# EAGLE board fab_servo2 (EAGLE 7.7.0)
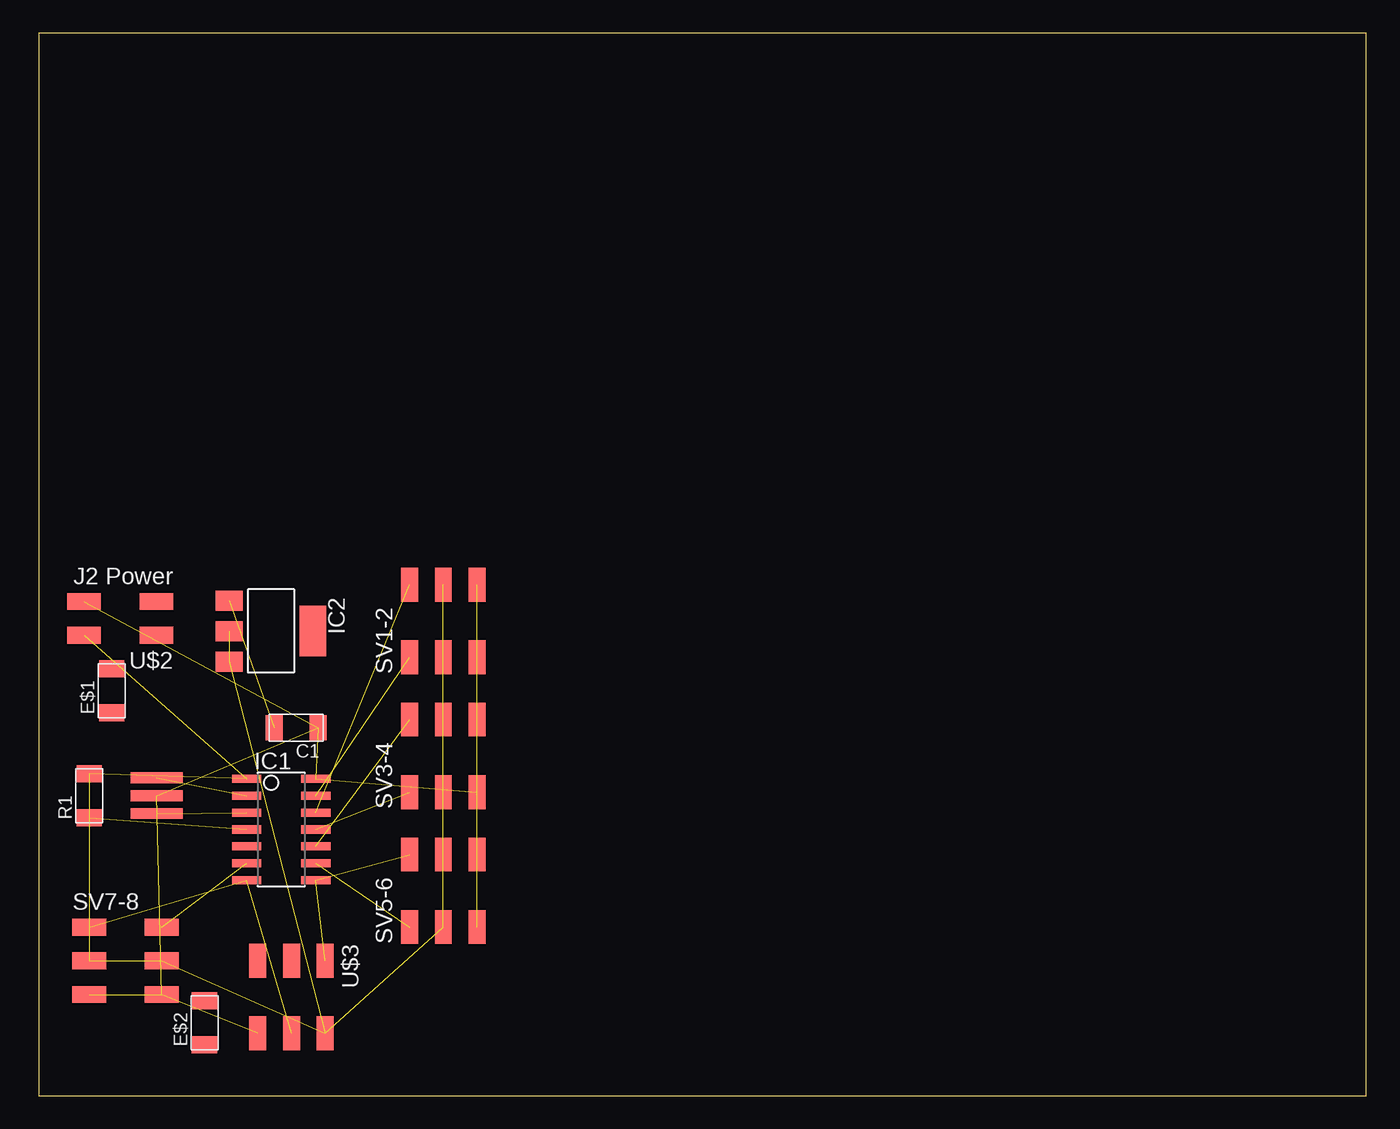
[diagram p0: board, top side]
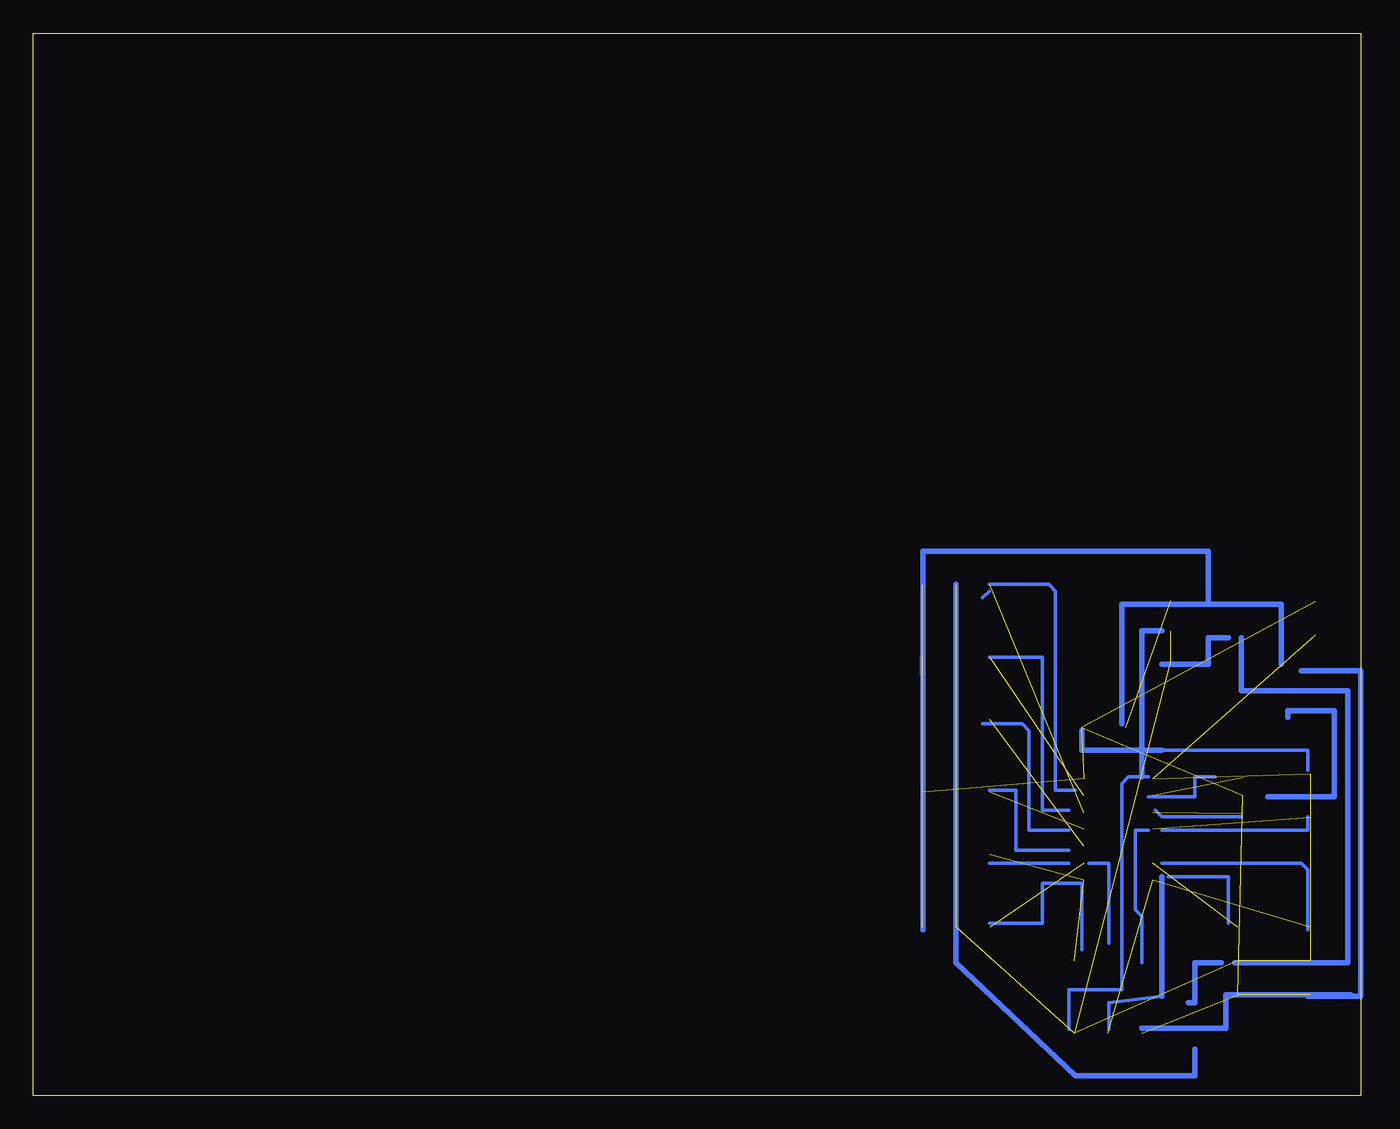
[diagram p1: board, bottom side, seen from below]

Size 100 x 80 mm. Coordinates in mm from the lower left corner, seen from the top.
Outline: 0,0 100,0 100,80 0,80 0,0
Copper layers (1*16): Top 0.035mm / dielectric 1.5mm / Bottom 0.035mm
Design rules "default": minimum track width 10mil, minimum drill 24mil, track to track 8mil, track to pad 8mil, pad to pad 8mil, via to via 8mil, smd to smd 8mil, copper to edge 40mil, drill to drill 8mil, minimum pad ring 10mil, minimum via ring 8mil, stop-mask expansion 4mil, vias tented up to drill 0mil, thermal gap 10mil

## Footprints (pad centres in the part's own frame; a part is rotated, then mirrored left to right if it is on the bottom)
C1206FAB = smd 1.27 x 1.905: 1 -1.651,0; 2 1.651,0
R1206FAB = smd 1.27 x 1.905: 1 -1.651,0; 2 1.651,0
SOIC14 = smd 0.61 x 2.21: 1 -3.81,-2.603; 2 -2.54,-2.603; 3 -1.27,-2.603; 4 0,-2.603; 5 1.27,-2.603; 6 2.54,-2.603; 7 3.81,-2.603; 8 3.81,2.603; 9 2.54,2.603; 10 1.27,2.603; 11 0,2.603; 12 -1.27,2.603; 13 -2.54,2.603; 14 -3.81,2.603
SOT223 = smd 1.499 x 2.007: 1 -2.261,-3.15; 2 0.025,-3.15; 3 2.311,-3.15 | smd 3.81 x 2.007: 4 0,3.15
2X03SMD = smd 2.54 x 1.27: 1 -2.54,2.54; 2 2.92,2.54; 3 -2.54,0; 4 2.92,0; 5 -2.54,-2.54; 6 2.92,-2.54
EFOBM = smd 0.8 x 3.9: 1 -1.35,0; 2 0,0; 3 1.35,0
2X02SMD = smd 2.54 x 1.27: 1 -2.54,1.27; 2 2.92,1.27; 3 -2.54,-1.27; 4 2.92,-1.27

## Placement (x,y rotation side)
C1  22μF  [C1206FAB]  19.39,27.71 180 top
E$1  [R1206FAB]  5.5,30.5 90 top
E$2  [R1206FAB]  12.5,5.5 90 top
IC1  ATTINY44-SSU  [SOIC14]  18.28,20.05 270 top
IC2  REG1117  [SOT223]  17.5,35 270 top
R1  10k  [R1206FAB]  3.81,22.59 90 top
SV1-2  [2X03SMD]  30.48,35.56 90 top
SV3-4  [2X03SMD]  30.48,25.4 90 top
SV5-6  [2X03SMD]  30.48,15.24 90 top
SV7-8  [2X03SMD]  6.35,10.16 0 top
U$1  20MHz  [EFOBM]  8.89,22.59 270 top
U$2  J2 Power  [2X02SMD]  6.34,35.94 180 top
U$3  AVRISPSMD  [2X03SMD]  19.05,7.62 270 top

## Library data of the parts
C1 E$1 E$2 IC1 R1 SV1-2 SV3-4 SV5-6 SV7-8 U$1-U$3 = fab
IC2 = burr-brown; MPN: REG1117; OC_FARNELL: 1097566; OC_NEWARK: 14P6981

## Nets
GND: C1.1 IC1.14 SV1-2.5 SV1-2.6 SV3-4.5 SV3-4.6 SV5-6.5 SV5-6.6 SV7-8.5 SV7-8.6 U$1.2 U$2.4 U$3.6
N$1: IC1.7 SV7-8.1 U$3.4
N$2: IC1.4 R1.1
N$3: IC1.6 SV7-8.2
N$4: IC1.3 U$1.3
N$5: IC1.2 U$1.1
N$6: IC1.13 SV1-2.1
N$7: IC1.12 SV1-2.2
N$8: IC1.11 SV3-4.1
N$9: IC1.10 SV3-4.2
N$10: IC1.9 SV5-6.1
N$11: IC1.8 SV5-6.2 U$3.1
N$39: C1.2 IC2.1
VCC: IC1.1 IC2.2 IC2.3 R1.2 SV1-2.3 SV1-2.4 SV3-4.3 SV3-4.4 SV5-6.3 SV5-6.4 SV7-8.3 SV7-8.4 U$2.2 U$3.2

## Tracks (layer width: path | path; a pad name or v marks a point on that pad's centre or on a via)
GND  (12 unrouted)
N$1  (2 unrouted)
N$2  (1 unrouted)
N$3  (1 unrouted)
N$4  (1 unrouted)
N$5  (1 unrouted)
N$6  (1 unrouted)
N$7  (1 unrouted)
N$8  (1 unrouted)
N$9  (1 unrouted)
N$10  (1 unrouted)
N$11  (2 unrouted)
N$12
  Bottom 0.254: 19,11.5 19,17.5 20.5,17.5
N$13
  Bottom 0.406: 0.77,7.62 10.16,7.62 10.16,5.08 16.51,5.08
N$14
  Bottom 0.254: 16,24 16.5,24 17.5,24 18,23.5 18,8 22,8 22,5 | 4,24.5 4,26 15,26 15.5,26
  Bottom 0.406: 15,35 16.5,35 16.5,26 | 16.5,26 16.5,24 | 16.5,26 15,26 | 16.5,26 21,26 21,27.5
N$16
  Bottom 0.254: 15,15.5 15,7.5 19,7 19,5
  Bottom 0.406: 15,7.5 15,16.5
N$17
  Bottom 0.406: 10,34.5 11.5,34.5 11.5,32.5 15,32.5
N$18
  Bottom 0.254: 16.5,10 16.5,13.5 17,14 17,20 16,20
N$19
  Bottom 0.254: 9,21 15,21 15.5,21.5
N$20
  Bottom 0.406: 33.02,31.75 33.02,33.02
N$21
  Bottom 0.254: 11,24 12.5,24 12.5,22.5 16,22.5
N$22
  Bottom 0.406: 7,22.5 2,22.5 2,29 5.5,29 5.5,28.5
N$23
  Bottom 0.406: 9.5,10 1,10 1,30.5 9,30.5 9,34.5
N$25
  Bottom 0.254: 15,20 4,20 4,21
N$27
  Bottom 0.254: 14.5,16.5 10,16.5 10,13
N$28
  Bottom 0.254: 15,17.5 4.5,17.5 4,17 4,12.5
N$29
  Bottom 0.254: 21,11 21,16 24,16 24,13 28,13
N$30
  Bottom 0.254: 21.5,23 23,23 23,38 23.5,38.5 28,38.5
N$31
  Bottom 0.254: 22,21.5 24,21.5 24,33 28,33
N$32
  Bottom 0.254: 22,20 25,20 25,27.5 25.5,28 28.5,28
N$33
  Bottom 0.254: 22,18.5 26,18.5 26,23 28,23
N$34
  Bottom 0.254: 28,38 28.5,37.5
N$35
  Bottom 0.254: 22,17.5 28,17.5
N$36
  Bottom 0.254: 30.5,12.5 30.5,12
  Bottom 0.406: 30.5,38.5 30.5,12.5 30.5,10 21.5,1.5 12.5,1.5 12.5,3.5
N$39  (1 unrouted)
S$1
  Bottom 0.254: 33,12.5 33,13
  Bottom 0.406: 33,12.5 33,41 11.5,41 11.5,37 | 18,28 18,37 11.5,37 | 11.5,37 6,37 6,32.5
S$2
  Bottom 0.406: 10.5,10 12.5,10 12.5,7 13,7
S$3
  Bottom 0.406: 4.5,32 0,32 0,7.5 4,7.5
VCC  (13 unrouted)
